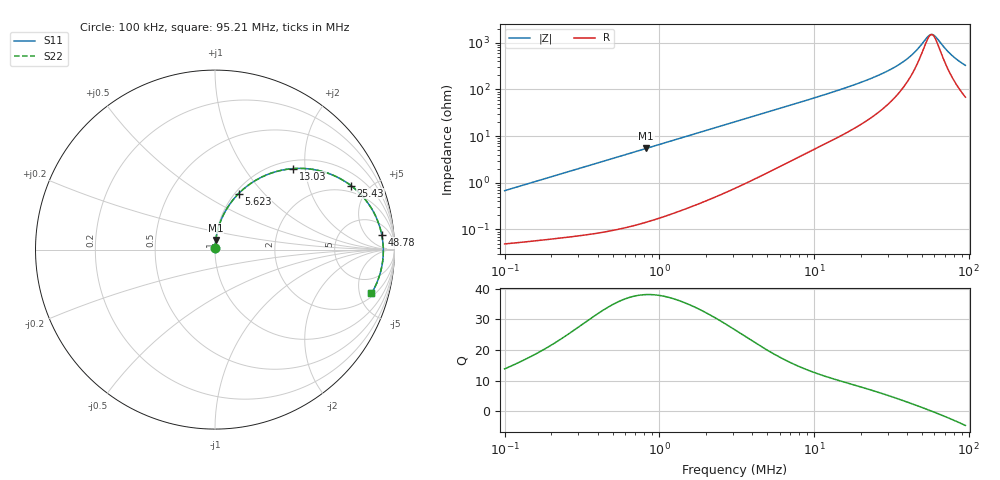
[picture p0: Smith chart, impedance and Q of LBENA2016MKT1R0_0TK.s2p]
! LBENA2016MKT1R0_0TK  S-PARAMETER MODEL  ( Standard Model )
! Model Generated by TAIYO YUDEN Corporation (http://www.ty-top.com)
! Version 1.0
! TAIYO YUDEN Control No. 20240828
! Copyright(c) 2024 TAIYO YUDEN CO.,LTD. All Rights Reserved.
! Product Description (link to TY-COMPAS)
! https://ds.yuden.co.jp/TYCOMPAS/or/detail?pn=LBENA2016MKT1R0M0TK&u=M
! Products Name : Inductors
! Characteristics :
!  Inductance : 1.0 [uH] , SRF(min) : - [Hz] , DC Resistance(max) : 0.045 [Ohm]
!  Rated Current : Saturation  3100 [mA] , Temp Rise  3200 [mA] (40 [degC])
!  Case Size : 2.0 x 1.6 / 0.079 x 0.063 [mm/inch] , Thickness : 1.2 / 0.047 [mm/inch]
!  (Conditions: Temperature = 25 [degC] , DC Bias Current = 0 [A])
! External Node Assignments :
!  1  o---GGG---o  2
! GND o---------o GND
! Frequency Range : 0.1MHz  -  95.211795MHz  [ 402 STEP ]
# MHz S RI R 50
! Freq[MHz].  S11 Real  S11 Imag  S21 Real  S21 Imag  S12 Real  S12 Imag  S22 Real  S22 Imag
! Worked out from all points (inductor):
!   401 points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, 100 kHz to 95.21 MHz, reference 50 ohm
!   read as one part in series: L = 1.07 uH near 103.5 kHz
!   highest Q = 38.1 at 824 kHz (marker M1), where L = 1.05 uH
!   self-resonance near 57.53 MHz
!   S11 on the Smith chart (normalised r, x): 100 kHz: 1.00, +0.01; 5.623 MHz: 1.04, +0.73; 13.03 MHz: 1.16, +1.72; 25.43 MHz: 1.61, +3.83; 48.78 MHz: 11, +14; 95.21 MHz: 2.37, -6.42
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0.1  0.000536 0.00676  0.9995 -0.00676  0.9995 -0.00676  0.000536 0.00676
0.31545  0.00119 0.021  0.9988 -0.021  0.9988 -0.021  0.00119 0.021
0.824038  0.00438 0.0542  0.9956 -0.0542  0.9956 -0.0542  0.00438 0.0542
0.995088  0.00602 0.0653  0.994 -0.0653  0.994 -0.0653  0.00602 0.0653
3.085641  0.0459 0.1913  0.9541 -0.1913  0.9541 -0.1913  0.0459 0.1913
5.623165  0.1319 0.3123  0.8681 -0.3123  0.8681 -0.3123  0.1319 0.3123
9.733658  0.3035 0.4226  0.6965 -0.4226  0.6965 -0.4226  0.3035 0.4226
13.02778  0.4344 0.4512  0.5656 -0.4512  0.5656 -0.4512  0.4344 0.4512
18.04506  0.597 0.4357  0.403 -0.4357  0.403 -0.4357  0.597 0.4357
25.42686  0.7569 0.3571  0.2431 -0.3571  0.2431 -0.3571  0.7569 0.3571
30.70484  0.8282 0.29  0.1718 -0.29  0.1718 -0.29  0.8282 0.29
39.71071  0.8981 0.1795  0.1019 -0.1795  0.1019 -0.1795  0.8981 0.1795
44.01372  0.9165 0.1312  0.0835 -0.1312  0.0835 -0.1312  0.9165 0.1312
48.78299  0.9293 0.0815  0.0707 -0.0815  0.0707 -0.0815  0.9293 0.0815
55.00415  0.937 0.0223  0.063 -0.0223  0.063 -0.0223  0.937 0.0223
56.92315  0.9377 0.00526  0.0623 -0.00526  0.0623 -0.00526  0.9377 0.00526
58.9091  0.9379 -0.0118  0.0621 0.0118  0.0621 0.0118  0.9379 -0.0118
62.01869  0.9369 -0.0375  0.0631 0.0375  0.0631 0.0375  0.9369 -0.0375
69.92777  0.9289 -0.0971  0.0711 0.0971  0.0711 0.0971  0.9289 -0.0971
77.50505  0.9157 -0.1476  0.0843 0.1476  0.0843 0.1476  0.9157 -0.1476
87.38907  0.8929 -0.2049  0.1071 0.2049  0.1071 0.2049  0.8929 -0.2049
95.21179  0.8717 -0.2443  0.1283 0.2443  0.1283 0.2443  0.8717 -0.2443
